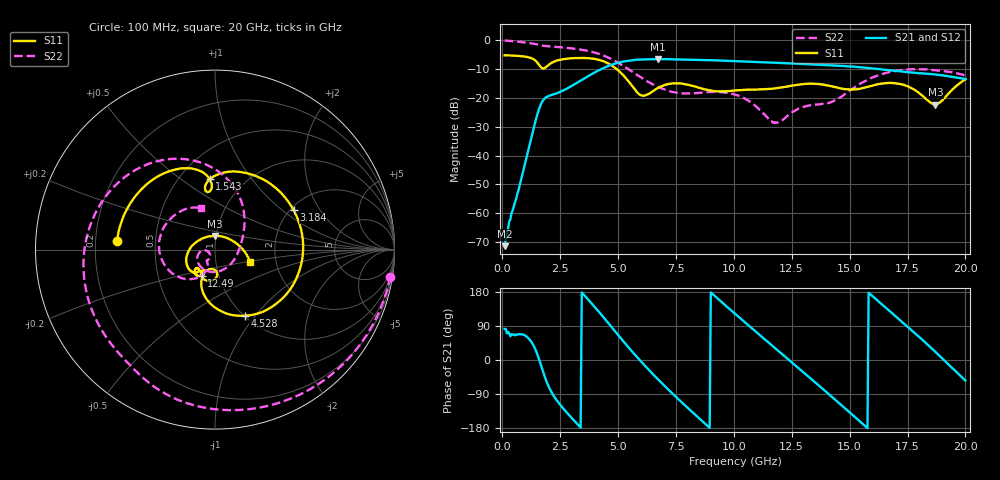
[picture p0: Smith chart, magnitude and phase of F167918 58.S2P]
!  2-Port S-parameters saved by WinCal
! VAR MeasName=S-Parameters (CALIBRATED_DATA) read from VNA (N5242A)
! VAR MeasDate=2016-11-22 10:27:40
! VAR NAME=F167918 58
! VAR FILENAME=F167918 58.S2P
! VAR DATE=2016-11-22 10:27:40
! VAR PHYS_PORTS=1,2
# Hz S DB R 50
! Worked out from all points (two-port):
!   401 points, 100 MHz to 20 GHz, reference 50 ohm
!   highest |S21| = -6.56 dB at 6.717 GHz (marker M1); lowest = -71.4 dB at 100 MHz (marker M2)
!   |S21| within 3 dB of the highest: 4.389 GHz to 15.73 GHz (11.34 GHz wide, 113 % of centre)
!   lowest |S11| = -22.3 dB at 18.71 GHz (marker M3), VSWR 1.17, Z = 49.5 + j7.62 ohm
!   |S11| at or under -10 dB: 4.938 GHz to end of sweep
!   |S22| runs from -28.7 to -0.1 dB; largest |S21 - S12| = 0.0037
!   S11 on the Smith chart (normalised r, x): 100 MHz: 0.29, +0.04; 1.543 GHz: 0.70, +0.65; 3.184 GHz: 2.09, +1.21; 4.528 GHz: 1.00, -0.88; 12.49 GHz: 0.83, -0.25; 20 GHz: 1.47, -0.22
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1e8  -5.23 174.9  -71.42 82.0  -71.47 70.2  -0.10 -8.8
8.4625e8  -5.58 136.0  -47.31 67.6  -47.23 68.0  -0.67 -67.2
1.54275e9  -8.09 94.3  -24.94 10.1  -24.95 10.2  -1.54 -113.3
1.84125e9  -9.63 99.0  -20.13 -45.4  -20.12 -45.4  -2.00 -128.9
2.3885e9  -6.99 77.0  -18.31 -109.2  -18.32 -109.3  -2.36 -155.4
3.1845e9  -6.19 26.6  -14.98 -165.3  -14.99 -165.2  -3.03 167.3
3.43325e9  -6.15 10.0  -13.78 178.2  -13.79 178.4  -3.34 155.8
4.52775e9  -7.88 -65.9  -9.10 101.2  -9.07 101.2  -5.85 103.5
5.72175e9  -16.97 -114.3  -6.85 14.3  -6.83 14.2  -11.54 52.7
6.71675e9  -16.62 -85.9  -6.56 -50.8  -6.57 -50.7  -16.17 17.0
6.7665e9  -16.42 -86.6  -6.57 -53.7  -6.57 -53.7  -16.36 14.8
7.61225e9  -14.96 -106.9  -6.64 -103.8  -6.65 -103.8  -18.29 -25.3
8.5575e9  -16.64 -121.4  -6.82 -157.2  -6.80 -157.2  -18.23 -78.7
1.005e10  -17.44 -116.1  -7.24 122.0  -7.24 122.1  -18.87 -149.3
1.169175e10  -16.80 -115.7  -7.78 36.0  -7.75 35.9  -28.62 -158.5
1.248775e10  -15.79 -117.2  -8.05 -5.5  -8.04 -5.6  -25.13 -122.2
1.338325e10  -15.12 -126.6  -8.40 -52.5  -8.36 -52.4  -22.49 -126.9
1.427875e10  -16.11 -135.4  -8.75 -99.5  -8.74 -99.6  -21.25 -118.6
1.527375e10  -17.05 -129.1  -9.27 -152.8  -9.24 -153.3  -16.06 -117.0
1.67165e10  -14.87 -142.9  -10.38 129.7  -10.41 129.6  -11.09 -154.4
1.87065e10  -22.32 89.6  -11.90 21.4  -11.90 21.4  -10.43 145.3
2e10  -13.57 -20.0  -13.44 -54.2  -13.38 -54.0  -12.31 108.9
